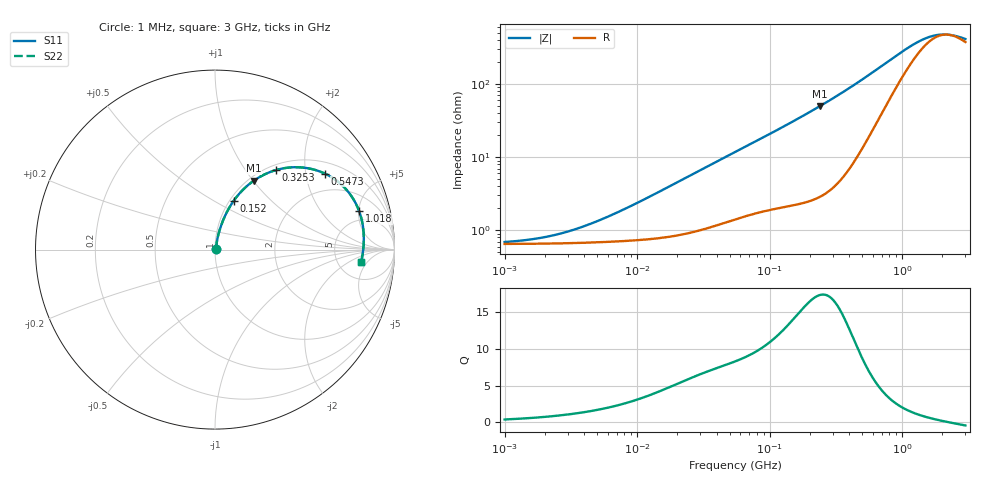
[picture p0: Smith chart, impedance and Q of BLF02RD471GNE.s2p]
! BLF02RD471GNE
# Hz S RI R 50
!Freq.(Hz) S11(Real) S11(Imag) S21(Real) S21(Imag) S12(Real) S12(Imag) S22(Real) S22(Imag)
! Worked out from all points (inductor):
!   401 points, 1 MHz to 3 GHz, reference 50 ohm
!   read as one part in series: L = 35.7 nH near 9.794 MHz
!   highest Q = 17.4 at 240.9 MHz (marker M1), where L = 33.2 nH
!   self-resonance near 2.219 GHz
!   S11 on the Smith chart (normalised r, x): 1 MHz: 1.01, +0.00; 152 MHz: 1.04, +0.62; 325.3 MHz: 1.09, +1.39; 547.3 MHz: 1.35, +2.57; 1.018 GHz: 3.62, +5.05; 3 GHz: 8.53, -3.46
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1000000  0.00649 0.00231  0.9935 -0.00231  0.9935 -0.00231  0.00649 0.00231
2014875  0.00657 0.00463  0.9934 -0.00463  0.9934 -0.00463  0.00657 0.00463
2775447  0.00665 0.00636  0.9934 -0.00636  0.9934 -0.00636  0.00665 0.00636
3823119  0.00678 0.0087  0.9932 -0.0087  0.9932 -0.0087  0.00678 0.0087
6831390  0.00723 0.0153  0.9928 -0.0153  0.9928 -0.0153  0.00723 0.0153
1.461624e7  0.00881 0.0322  0.9912 -0.0322  0.9912 -0.0322  0.00881 0.0322
3.00453e7  0.0142 0.0644  0.9858 -0.0644  0.9858 -0.0644  0.0142 0.0644
5.477226e7  0.0268 0.1121  0.9732 -0.1121  0.9732 -0.1121  0.0268 0.1121
9.402997e7  0.0529 0.1814  0.9471 -0.1814  0.9471 -0.1814  0.0529 0.1814
1.520175e8  0.1051 0.2734  0.8949 -0.2734  0.8949 -0.2734  0.1051 0.2734
2.094008e8  0.1728 0.3494  0.8272 -0.3494  0.8272 -0.3494  0.1728 0.3494
2.408952e8  0.2151 0.3832  0.7849 -0.3832  0.7849 -0.3832  0.2151 0.3832
3.252521e8  0.3376 0.4425  0.6624 -0.4425  0.6624 -0.4425  0.3376 0.4425
4.219165e8  0.4732 0.4584  0.5268 -0.4584  0.5268 -0.4584  0.4732 0.4584
5.473095e8  0.6117 0.4237  0.3883 -0.4237  0.3883 -0.4237  0.6117 0.4237
6.685918e8  0.6998 0.3662  0.3002 -0.3662  0.3002 -0.3662  0.6998 0.3662
8.005644e8  0.7571 0.3023  0.2429 -0.3023  0.2429 -0.3023  0.7571 0.3023
1.017911e9  0.8026 0.2157  0.1974 -0.2157  0.1974 -0.2157  0.8026 0.2157
1.402151e9  0.8261 0.1149  0.1739 -0.1149  0.1739 -0.1149  0.8261 0.1149
1.782824e9  0.8291 0.0516  0.1709 -0.0516  0.1709 -0.0516  0.8291 0.0516
2.266846e9  0.8254 -0.0049  0.1746 0.0049  0.1746 0.0049  0.8254 -0.0049
3e9  0.8145 -0.0674  0.1855 0.0674  0.1855 0.0674  0.8145 -0.0674
